PROGRAM MAIN
VAR
	bCONNECT: BOOL;
	bEXECUTE: BOOL;
	bREAD : BOOL;
	bDISCONNECT: BOOL;
	
	stRecordArr: ARRAY [1..20] OF ST_Record;
	nRecs: UDINT;		
	nRecordStartIndex: UDINT;
		
	R_TRIG1: R_TRIG;	
	R_TRIG2: R_TRIG;
	R_TRIG3: R_TRIG;
	R_TRIG4: R_TRIG;
		
	nState: INT;
	nState_Connect: INT;
	nState_Disconnect: INT;
	
	bConn: BOOL;
	bSP: BOOL;	
	bResult: BOOL;
	bData: BOOL;
		
	nDBID: UDINT := 1;
	
	fbSQLDatabase: FB_SQLDatabaseEvt(sNetID:='', tTimeout:=T#10S);
	fbSQLStoredProcedure: FB_SQLStoredProcedureEvt(sNetID:='', tTimeout:=T#10S);
	fbSQLResult: FB_SQLResultEvt(sNetID:='', tTimeout:=T#10S);
	
	arrParameter: ARRAY [0..0] OF ST_SQLSPParameter;
	
	nCustomerID: DINT := 12345;
	
	
	ipResultEvt : Tc3_Eventlogger.I_TcMessage;
	bError : BOOL;
	nEventID: UDINT;
	sEventClass : STRING(255);
	sEventMsg : STRING(255);
END_VAR

R_TRIG1(CLK:=bCONNECT);
IF R_TRIG1.Q AND nState = 0 THEN
	bCONNECT := FALSE;
	nState := 1;
END_IF	

R_TRIG2(CLK:=bEXECUTE);
IF R_TRIG2.Q AND nState = 0 THEN
	bEXECUTE := FALSE;
	nState := 2;
END_IF	

R_TRIG3(CLK:=bREAD);
IF R_TRIG3.Q AND nState = 0 THEN
	bREAD := FALSE; 
	nState := 3;
END_IF

R_TRIG4(CLK:=bDISCONNECT);
IF R_TRIG4.Q THEN
	bDISCONNECT := FALSE;
	nState := 4;
END_IF

CASE nState OF
	0:(*Idle*)
		;
	1: // Connect to database and create stored procedure instance 
		CASE nState_Connect OF
			0:
				IF fbSQLDatabase.Connect(hDBID:= nDBID) THEN
					ipResultEvt := fbSQLDatabase.ipTcResult;
					bConn := NOT fbSQLDatabase.bError;
					IF bConn THEN
						nState_Connect := 1;
					ELSE
						nState:=200;
					END_IF
				END_IF 
			1:
				arrParameter[0].sParameterName := '@Customer_ID';
				arrParameter[0].eParameterDataType := Tc3_Database.E_ColumnType.Integer;
				arrParameter[0].eParameterType := E_SPParameterType.Input;
				arrParameter[0].nParameterSize := SIZEOF(nCustomerID);
						
				IF fbSQLDatabase.CreateSP('SP_GetCustomerPositions', ADR(arrParameter), SIZEOF(arrParameter), ADR(fbSQLStoredProcedure)) THEN
					ipResultEvt := fbSQLDatabase.ipTcResult;
					bSP := NOT fbSQLDatabase.bError;
					nState_Connect:=0;
					nState := 200;					
				END_IF			
		END_CASE
	2: // Execute stored procedure
		IF fbSQLStoredProcedure.ExecuteDataReturn(pParameterStrc:= ADR(nCustomerID), cbParameterStrc:= SIZEOF(nCustomerID), pSQLDBResult:= ADR(fbSQLResult)) THEN
			ipResultEvt := fbSQLStoredProcedure.ipTcResult;
			MEMSET(ADR(stRecordArr),0,SIZEOF(stRecordArr));
			bResult := NOT fbSQLStoredProcedure.bError;
			nState := 200;			
		END_IF
	3:	// Read customer positions
		IF fbSQLResult.Read(nRecordStartIndex, 20, ADR(stRecordArr), SIZEOF(stRecordArr), TRUE, FALSE) THEN
			ipResultEvt := fbSQLResult.ipTcResult;
			bData := NOT fbSQLStoredProcedure.bError;
			nRecs := fbSQLResult.nDataCount;
			nState := 200;						
		END_IF
	4:// Disconnect all
		CASE nState_Disconnect OF
			0:
				IF bData THEN
					IF fbSQLResult.Release() THEN
						nState_Disconnect := 1;
					END_IF
				ELSE
					nState_Disconnect := 1;
				END_IF
			1:
				IF bSP THEN
					IF fbSQLStoredProcedure.Release() THEN
						nState_Disconnect := 2;
					END_IF
				ELSE
					nState_Disconnect := 2;
				END_IF
			2:
				IF bConn THEN
					IF fbSQLDatabase.Disconnect() THEN
						nState_Disconnect := 3;
					END_IF
				ELSE
					nState_Disconnect := 3;
				END_IF
			3:
				bData := FALSE;
				bSP := FALSE;
				bConn := FALSE;
				bResult := FALSE;
				sEventClass := '';
				sEventMsg := '';
				nEventID := 0;
				bError := FALSE;
				nState_Disconnect := 0;
				nState := 0;
		END_CASE
	200:	 
        IF ipResultEvt.RequestEventText(1033, sEventMsg, SIZEOF(sEventMsg)) THEN
            nState := 201;
        END_IF
	201:
        IF ipResultEvt.RequestEventClassName(1033, sEventClass, SIZEOF(sEventClass)) THEN
            
            nEventID := ipResultEvt.nEventId;

            bError := (ipResultEvt.eSeverity = TcEventSeverity.Error) OR
                     (ipResultEvt.eSeverity = TcEventSeverity.Critical);

            nState:=0;                     
        END_IF		
END_CASE

END_PROGRAM
